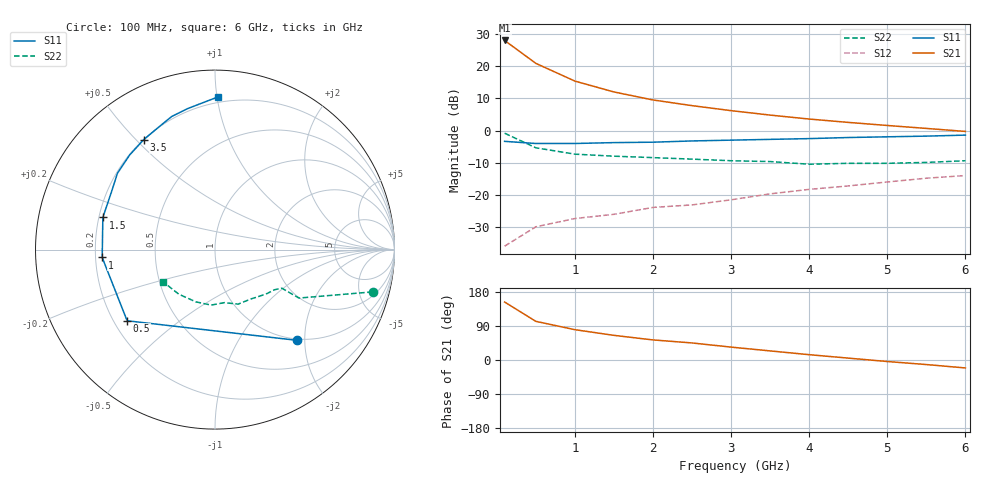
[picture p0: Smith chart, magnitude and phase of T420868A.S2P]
! AT-42086
!S AND NOISE PARAMETERS at Vce=8V  Ic=10mA.  LAST UPDATED 07-21-92
# ghz s ma r 50
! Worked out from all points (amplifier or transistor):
!   13 points, 100 MHz to 6 GHz, reference 50 ohm
!   highest |S21| = 28.0 dB at 100 MHz (marker M1)
!   |S21| within 3 dB of that: start of sweep to 268.6 MHz
!   unconditionally stable (mu >= 1): 1.333 GHz to 3.696 GHz
!   at 1 GHz: K = 0.87, MSG = 21.4 dB, |S12| = -27.3 dB
!   at 3 GHz: K = 1.13, MAG = 11.7 dB, |S12| = -21.5 dB
!   at 6 GHz: K = 0.65, MSG = 6.9 dB, |S12| = -14.0 dB
!   lowest NFmin = 1.00 dB at 100 MHz
!   S11 on the Smith chart (normalised r, x): 100 MHz: 0.97, -1.83; 500 MHz: 0.25, -0.33; 1 GHz: 0.23, -0.03; 1.5 GHz: 0.22, +0.13; 3.5 GHz: 0.20, +0.53; 6 GHz: 0.16, +1.00
0.1  0.68 -48.0  25.12 153.0  0.016 65.0  0.91 -15.0
0.5  0.63 -141.0  11.07 102.0  0.032 42.0  0.54 -30.0
1  0.63 -176.0  5.87 80.0  0.043 43.0  0.43 -30.0
1.5  0.65 164.0  3.98 65.0  0.05 46.0  0.4 -34.0
2  0.66 151.0  2.99 53.0  0.064 52.0  0.38 -40.0
2.5  0.69 142.0  2.44 45.0  0.07 53.0  0.36 -46.0
3  0.71 132.0  2.04 34.0  0.084 54.0  0.34 -54.0
3.5  0.73 123.0  1.74 24.0  0.104 53.0  0.33 -67.0
4  0.75 115.0  1.51 14.0  0.122 51.0  0.3 -80.0
4.5  0.78 108.0  1.34 5.0  0.138 50.0  0.31 -94.0
5  0.8 101.0  1.2 -4.0  0.159 46.0  0.31 -110.0
5.5  0.82 95.0  1.08 -12.0  0.182 40.0  0.32 -129.0
6  0.85 89.0  0.97 -21.0  0.2 35.0  0.34 -148.0
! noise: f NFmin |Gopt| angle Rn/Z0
0.1  1  0.04  8  0.13
0.5  1.1  0.03  62  0.12
1  1.5  0.06  168  0.12
2  1.9  0.25  -146  0.12
4  3.5  0.58  -100  0.52
